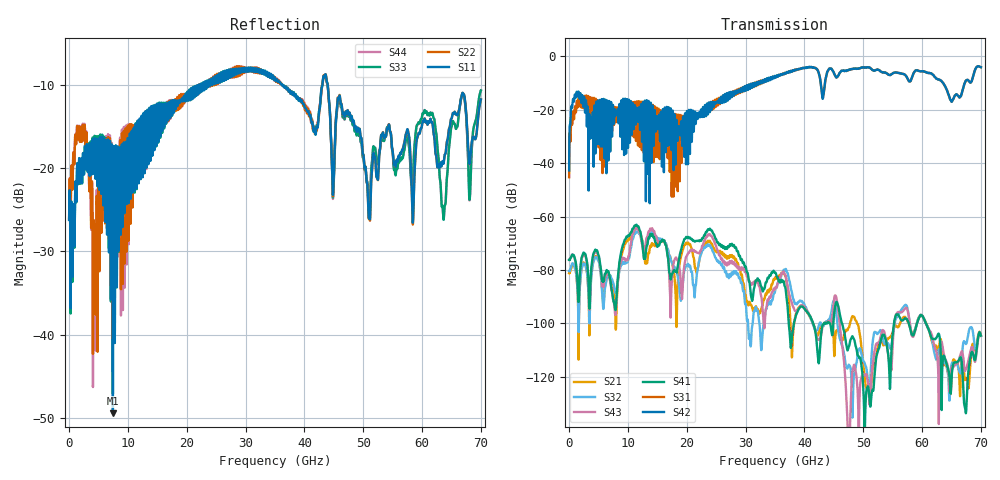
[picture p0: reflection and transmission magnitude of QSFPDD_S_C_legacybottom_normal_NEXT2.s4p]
! AWR Design Environment (8415) Thu Dec 20 15:14:50 2018
! Document = 'CHANNEL TEST'
! nPorts: 4, nXvals: 7001
# HZ S DB R 50
!Freq DBS11 AngS11 DBS12 AngS12 DBS13 AngS13 DBS14 AngS14
!	DBS21 AngS21 DBS22 AngS22 DBS23 AngS23 DBS24 AngS24
!	DBS31 AngS31 DBS32 AngS32 DBS33 AngS33 DBS34 AngS34
!	DBS41 AngS41 DBS42 AngS42 DBS43 AngS43 DBS44 AngS44
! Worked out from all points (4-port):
!   7000 points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, 10 MHz to 70 GHz, reference 50 ohm
!   strongest paths, dB at 10 MHz, 17.51 GHz, 35.01 GHz, 52.51 GHz, 70 GHz:
!     S42: -42.7, -23.6, -7.5, -5.0, -4.0
!     S31: -45.3, -28.7, -7.5, -5.0, -4.0
!     S41: -76.2, -81.5, -81.0, -110.1, -104.6
!     S43: -76.2, -82.9, -87.1, -107.2, -104.7
!     S32: -80.5, -77.4, -88.0, -103.7, -104.6
!     S21: -81.2, -77.3, -83.1, -108.7, -104.5
!   lowest |S11| = -49.4 dB at 7.45 GHz (marker M1), VSWR 1.01, Z = 50.3 + j0.0931 ohm
!   |S11| at or under -10 dB: start of sweep to 22.1 GHz; 36.25 GHz to 43.06 GHz (6.813 GHz wide, 17.2 % of centre); 43.96 GHz to end of sweep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
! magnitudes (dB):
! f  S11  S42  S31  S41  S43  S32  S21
! 10 MHz  -26.2  -42.7  -45.3  -76.2  -76.2  -80.5  -81.2
! 1.29 GHz  -22.3  -13.2  -17.1  -80.0  -80.2  -83.0  -83.2
! 7.45 GHz  -49.4  -18.2  -18.5  -90.3  -90.5  -84.4  -86.0
! 11.41 GHz  -16.6  -22.2  -26.3  -63.1  -64.1  -65.6  -64.4
! 17.34 GHz  -11.9  -21.5  -22.6  -83.0  -90.9  -76.6  -76.4
! 23.89 GHz  -9.6  -20.4  -18.6  -64.6  -66.6  -70.6  -69.1
! 70 GHz  -11.8  -4.0  -4.0  -104.6  -104.7  -104.6  -104.5
